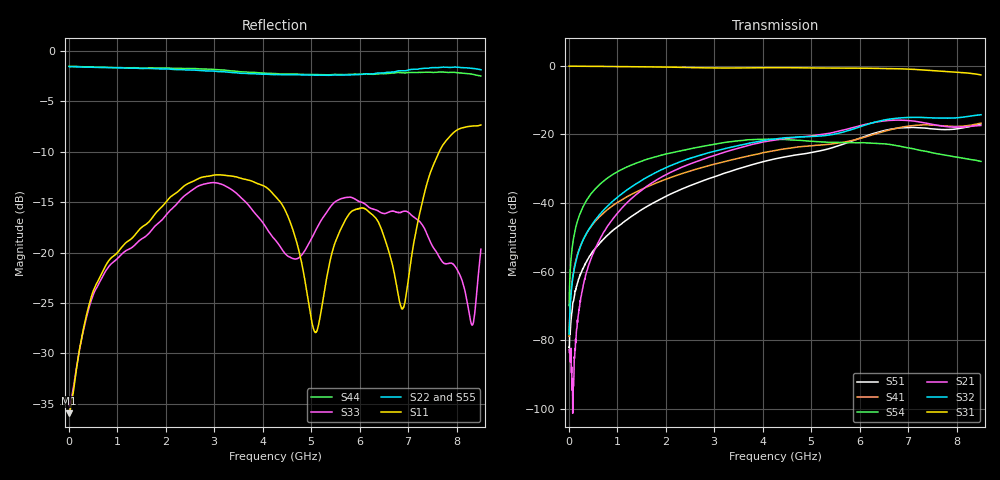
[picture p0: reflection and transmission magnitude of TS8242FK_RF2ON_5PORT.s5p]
! Created with skrf (http://scikit-rf.org).
# Hz S RI R 50.0
!freq ReS11 ImS11 ReS12 ImS12 ReS13 ImS13
! ReS14 ImS14 ReS15 ImS15
! ReS21 ImS21 ReS22 ImS22 ReS23 ImS23
! ReS24 ImS24 ReS25 ImS25
! ReS31 ImS31 ReS32 ImS32 ReS33 ImS33
! ReS34 ImS34 ReS35 ImS35
! ReS41 ImS41 ReS42 ImS42 ReS43 ImS43
! ReS44 ImS44 ReS45 ImS45
! ReS51 ImS51 ReS52 ImS52 ReS53 ImS53
! ReS54 ImS54 ReS55 ImS55
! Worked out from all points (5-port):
!   1601 points, 10 MHz to 8.5 GHz, reference 50 ohm
!   strongest paths, dB at 10 MHz, 2.132 GHz, 4.255 GHz, 6.378 GHz, 8.5 GHz:
!     S31: -0.2, -0.5, -0.6, -0.8, -2.7
!     S32: -78.2, -29.0, -21.4, -16.2, -14.3
!     S21: -82.7, -30.9, -21.7, -16.4, -17.5
!     S54: -69.9, -25.4, -21.5, -22.7, -27.9
!     S41: -78.8, -32.5, -24.8, -19.7, -16.8
!     S51: -82.0, -37.2, -27.2, -19.4, -17.0
!   lowest |S11| = -36.0 dB at 10 MHz (marker M1), VSWR 1.03, Z = 51.6 - j0.12 ohm
!   |S11| at or under -10 dB: start of sweep to 7.64 GHz
